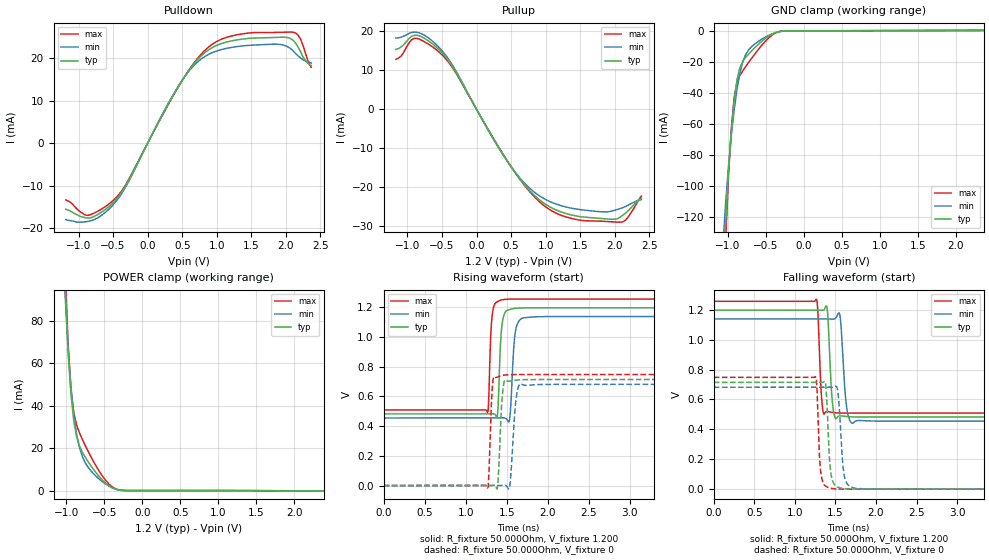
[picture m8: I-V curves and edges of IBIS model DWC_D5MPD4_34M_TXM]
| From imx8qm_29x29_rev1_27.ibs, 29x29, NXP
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[Model] DWC_D5MPD4_34M_TXM
Model_type   I/O
Polarity   Non-Inverting
Enable   Active-High
C_comp   1.453pF   1.359pF   1.567pF
C_comp_pullup   324.720fF   303.353fF   351.193fF
C_comp_pulldown 1.095pF   1.013pF   1.192pF
Vinh = 693.000mV
Vinl = 507.000mV
Vmeas = 600.000mV
Vref = 600.000mV
Rref = 50Ohms
Cref = 0pF
[Model Spec]
Vinh   693.000mV   663.000mV   723.000mV
Vinl   507.000mV   477.000mV   537.000mV
Vmeas   600.000mV   570.000mV   630.000mV
Vref   600.000mV   570.000mV   630.000mV
D_overshoot_ampl_h 0.4 NA   NA
D_overshoot_ampl_l 0.4 NA   NA
D_overshoot_area_l 60.000p NA   NA
D_overshoot_area_h 60.000p NA   NA
[Receiver Thresholds]
Vcross_low = 480.000mV
Vcross_high = 720.000mV
Vdiff_ac = 136.000mV
Vdiff_dc = 136.000mV
Tdiffslew_ac = 10.000ns
[Temperature Range]   25.000   125.000   -40.000
[Voltage Range]   1.200V   1.140V   1.260V
[GND Clamp Reference]   0.00V   0.00V   0.00V
[C Comp Corner]
| variable   typ   min   max
C_comp 1.453pF   1.567pF   1.359pF
C_comp_pullup 324.720fF   351.193fF   303.353fF
C_comp_pulldown 1.095pF   1.192pF   1.013pF
[Pulldown Reference]   0.00V   0.00V   0.00V
[POWER Clamp Reference]   1.200V   1.140V   1.260V
[Pullup Reference]   1.200V   1.140V   1.260V
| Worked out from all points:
|   slope of the pulldown table from 0 to 0.18 V, typ, clamps not added: 32 ohm
|   slope of the pullup table from 0 to 0.18 V, typ, clamps not added: 32.1 ohm
|   GND clamp passes 1 mA (typ) near -0.36 V on its own axis
|   POWER clamp passes 1 mA (typ) near -0.38 V on its own axis
|   rising waveform, R_fixture 50.000Ohm, V_fixture 1.200: 20-80 % time 35ps typ, 42.7ps min, 30.5ps max; typ from 0.482 V to 1.2 V
|   rising waveform, R_fixture 50.000Ohm, V_fixture 0: 20-80 % time 36.7ps typ, 48.2ps min, 30.2ps max; typ from 0 V to 0.714 V
|   falling waveform, R_fixture 50.000Ohm, V_fixture 1.200: 20-80 % time 39.6ps typ, 49.6ps min, 33.4ps max; typ from 1.2 V to 0.482 V
|   falling waveform, R_fixture 50.000Ohm, V_fixture 0: 20-80 % time 40.6ps typ, 49.6ps min, 34.5ps max; typ from 0.714 V to 0 V
[GND Clamp]
-1.184V   -348.5mA   -259.9mA   -439.9mA
-1.069V   -169.5mA   -142.4mA   -196.8mA
-1.031V   -126.4mA   -112.9mA   -139.4mA
-954.5mV  -65.34mA   -67.95mA   -63.85mA
-916.4mV  -45.2mA    -51.17mA   -43.27mA
-878.2mV  -31.45mA   -37.57mA   -33.15mA
-840mV    -23.64mA   -27.11mA   -28.67mA
-763.6mV  -17.03mA   -15.11mA   -22.94mA
-610.9mV  -9.282mA   -7.243mA   -12.78mA
-420mV    -2.151mA   -2.011mA   -2.842mA
-267.3mV  -90.01uA   -209.5uA   -60.56uA
2.367V    273.5uA    222.3uA    340.9uA
[Power Clamp]
-1.167V   319.3mA    247.1mA    390.6mA
-1.015V   97.56mA    92.13mA    106.5mA
-976.4mV  66.14mA    67.19mA    69.94mA
-938.2mV  45.51mA    48.6mA     48.18mA
-900mV    32.73mA    35.4mA     36.58mA
-861.8mV  25.19mA    26.24mA    30.62mA
-823.6mV  20.79mA    20mA       26.94mA
-747.3mV  15.56mA    12.93mA    21.03mA
-518.2mV  4.741mA    4.028mA    6.547mA
-403.6mV  1.468mA    1.527mA    1.973mA
-250.9mV  45.67uA    138.5uA    40.26uA
2.384V    -136.7uA   -117uA     -161.8uA
[Pulldown]
-1.184V   -15.5mA    -17.9mA    -13.3mA
-878.2mV  -17.54mA   -18.38mA   -16.95mA
-687.3mV  -16.38mA   -17.15mA   -15.65mA
-458.2mV  -13.22mA   -13.66mA   -12.79mA
-305.5mV  -9.62mA    -9.919mA   -9.404mA
496.4mV   14.65mA    14.67mA    14.62mA
725.5mV   19.66mA    19.09mA    19.97mA
992.7mV   22.9mA     21.6mA     23.8mA
1.871V    24.83mA    23.23mA    26mA
2.138V    23.55mA    21.09mA    25.9mA
2.215V    21.39mA    20mA       24.34mA
2.367V    18.2mA     18.8mA     17.8mA
[Pullup]
-1.167V   15.4mA     18.3mA     12.83mA
-900mV    19mA       19.82mA    18.23mA
-518.2mV  14.89mA    15.42mA    14.3mA
-327.3mV  10.4mA     10.72mA    10.12mA
207.3mV   -6.428mA   -6.573mA   -6.35mA
512.7mV   -15.06mA   -15.04mA   -15.05mA
780mV     -21.06mA   -20.42mA   -21.36mA
1.085V    -25.26mA   -23.84mA   -26.01mA
1.544V    -27.62mA   -25.82mA   -28.54mA
2.002V    -28.2mA    -25.86mA   -28.9mA
2.116V    -27.14mA   -25.21mA   -28.86mA
2.384V    -22.8mA    -23.14mA   -22.26mA
[Ramp]
R_load=50.000Ohm
dV/dt_r   428.700mV/37.000ps  409.289mV/45.500ps  448.470mV/31.000ps
dV/dt_f   428.700mV/41.000ps  409.289mV/50.500ps  448.470mV/34.500ps
[Rising waveform]
R_fixture=50.000Ohm
V_fixture=1.200
V_fixture_min=1.140
V_fixture_max=1.260
0s        482.4mV    455.1mV    509mV
1.263ns   482.4mV    455.1mV    492.1mV
1.313ns   482.7mV    455.1mV    1.096V
1.383ns   459.5mV    455mV      1.237V
1.434ns   1.046V     456mV      1.25V
1.474ns   1.16V      455.2mV    1.254V
1.534ns   1.185V     443.3mV    1.256V
1.604ns   1.193V     1.035V     1.256V
1.704ns   1.197V     1.13V      1.256V
10ns      1.197V     1.138V     1.256V
[Rising waveform]
R_fixture=50.000Ohm
V_fixture=0
0s        167nV      4.154uV    20.75nV
1.263ns   -3.174uV   -484.3nV   -16.41mV
1.323ns   759uV      17.44uV    657.8mV
1.383ns   -23.17mV   -105.4uV   729.8mV
1.434ns   519.1mV    604.1uV    740mV
1.474ns   709.4mV    1.558mV    744.3mV
1.534ns   702.7mV    -12.31mV   746.7mV
1.604ns   709.6mV    539.5mV    747.5mV
1.664ns   712.5mV    686.2mV    747.6mV
10ns      714mV      681.4mV    747.4mV
[Falling waveform]
R_fixture=50.000Ohm
V_fixture=1.200
V_fixture_min=1.140
V_fixture_max=1.260
0s        1.197V     1.138V     1.256V
1.263ns   1.197V     1.138V     1.271V
1.353ns   1.197V     1.138V     502.5mV
1.403ns   1.182V     1.138V     519.2mV
1.454ns   633.6mV    1.137V     513.5mV
1.504ns   470.6mV    1.145V     510.4mV
1.554ns   490.1mV    1.167V     509.3mV
1.634ns   485.5mV    564.1mV    508.7mV
1.704ns   483.3mV    440.7mV    508.6mV
10ns      482.4mV    455.1mV    508.9mV
[Falling waveform]
R_fixture=50.000Ohm
V_fixture=0
0s        714mV      681.4mV    747.3mV
1.263ns   714mV      681.4mV    747.3mV
1.323ns   713.6mV    681.4mV    95.82mV
1.383ns   683.7mV    681.4mV    18.64mV
1.423ns   231.6mV    681.1mV    8.903mV
1.464ns   56.18mV    681.6mV    3.864mV
1.534ns   11.87mV    632.8mV    910.7uV
1.614ns   3.701mV    76.84mV    187uV
1.734ns   517.6uV    6.505mV    35.32uV
10ns      492.3nV    4.285uV    122.5nV
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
